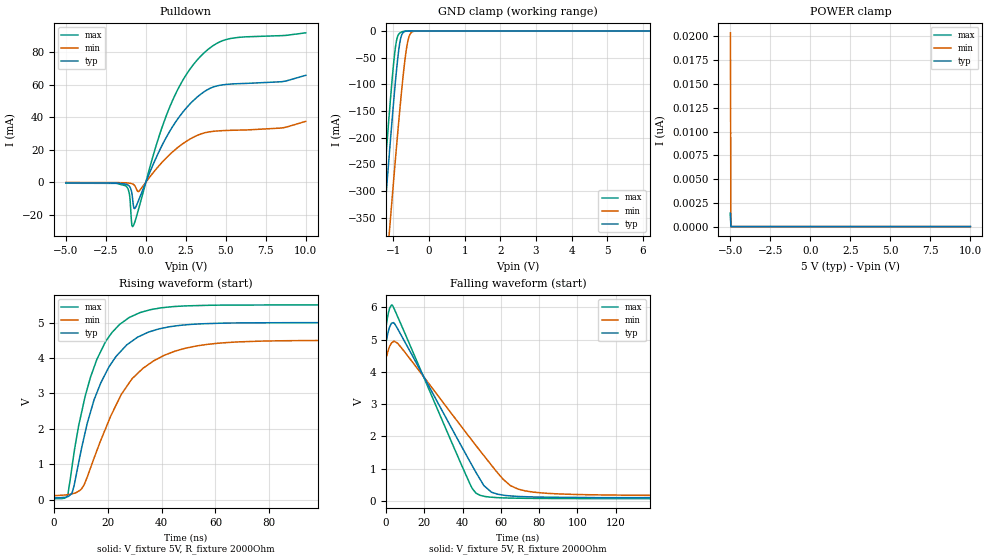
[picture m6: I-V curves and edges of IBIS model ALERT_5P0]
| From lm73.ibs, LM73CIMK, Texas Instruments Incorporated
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|   Model ALERT_5P0
[Model]   ALERT_5P0
Model_type   Open_drain
Polarity   Non-Inverting
Vmeas = 2.5
Vref = 5
Cref = 1pF
Rref = 2000
|   typ   min   max
|   (nom PVT)   (fast PVT)   (slow PVT)
C_comp   0.602p   0.543p   0.661p
|C_comp (ON state)   0.733p   0.730p   0.750p
|C_comp (OFF state)   0.602p   0.543p   0.661p
[Voltage Range]   5   4.5   5.5
[Temperature Range]   27   150   -40
[Pullup Reference]   5   4.5   5.5
[Pulldown Reference]   0   0   0
[Power Clamp Reference]   5   4.5   5.5
[GND Clamp Reference]   0   0   0
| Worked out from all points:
|   slope of the pulldown table from 0 to 0.75 V, typ, clamps not added: 43.3 ohm
|   GND clamp passes 1 mA (typ) near -0.68 V on its own axis
|   falling waveform, V_fixture 5V, R_fixture 2000Ohm: 20-80 % time 27ns typ, 33.7ns min, 23.6ns max; typ from 5 V to 0.097 V
|   rising waveform, V_fixture 5V, R_fixture 2000Ohm: 20-80 % time 13.6ns typ, 17.8ns min, 11.7ns max; typ from 0.097 V to 5 V
[Pulldown]
|   Voltage   I(typ)   I(min)   I(max)
-5V       -394uA     -141.8uA   -589.2uA
-1.25V    -1.146mA   -337.7uA   -2.189mA
-1.025V   -2.466mA   -540.2uA   -7.273mA
-890mV    -5.802mA   -809.4uA   -24.79mA
-815mV    -11.12mA   -1.087mA   -27.23mA
-665mV    -15.89mA   -2.513mA   -23.81mA
-425mV    -10.48mA   -5.487mA   -15.58mA
1.315V    28.32mA    15.36mA    41.94mA
2.32V     43.27mA    23.8mA     62.97mA
3.25V     52.8mA     29.03mA    75.76mA
5.05V     60.29mA    31.92mA    88mA
10V       65.91mA    37.54mA    92.06mA
[GND Clamp]
|   Voltage   I(typ)   I(min)   I(max)
-5V       -3.718A    -3.697A    -3.742A
-1.355V   -440.9mA   -580.8mA   -368mA
-1.25V    -349.5mA   -492.9mA   -274.4mA
-1.13V    -247.1mA   -393.7mA   -170.6mA
-1.07V    -197.3mA   -344.8mA   -121.2mA
-920mV    -81.51mA   -225.7mA   -22.09mA
-830mV    -27.93mA   -157.8mA   -4.69mA
-755mV    -6.077mA   -104.9mA   -1.502mA
-665mV    -667.7uA   -50.27mA   -221.1uA
-590mV    -95.28uA   -18.6mA    -27.79uA
-410mV    -439.3nA   -358.3uA   -36.45nA
10V       0A         0A         0A
[POWER Clamp]
|   Voltage   I(typ)   I(min)   I(max)
-5V       1.395nA    20.39nA    1.449nA
-4.97V    0A         0A         0A
-4.955V   0A         0A         0A
10V       0A         0A         0A
[Ramp]
R_load = 2000
|   typ   min   max
dV/dt_r   2.94209/1.35708e-08   2.60241/1.77746e-08   3.25792/1.17012e-08
dV/dt_f   2.94171/2.70212e-08   2.60108/3.36912e-08   3.2578/2.36341e-08
[Falling Waveform]
V_fixture = 5V
V_fixture_min = 4.5V
V_fixture_max = 5.5V
R_fixture = 2000Ohm
C_fixture = 0F
|   Time   V(typ)   V(min)   V(max)
0s        5V         4.5V       5.5V
1.801ns   5.386V     4.786V     5.966V
3.497ns   5.52V      4.927V     6.044V
8.162ns   5.106V     4.732V     5.423V
43.97ns   1.205V     1.949V     511.1mV
49.07ns   678.6mV    1.559V     176.5mV
55.11ns   269.9mV    1.105V     115.6mV
65ns      156.5mV    474.8mV    89.61mV
73ns      131.8mV    309.7mV    82.22mV
199.9ns   97.15mV    164.9mV    70.34mV
[Rising Waveform]
V_fixture = 5V
V_fixture_min = 4.5V
V_fixture_max = 5.5V
R_fixture = 2000Ohm
C_fixture = 0F
|   Time   V(typ)   V(min)   V(max)
0s        96.53mV    162.6mV    70.16mV
5.233ns   91.24mV    145mV      155.5mV
6.823ns   209.3mV    169.3mV    973.6mV
9.216ns   1.05V      244.2mV    2.089V
16ns      3.024V     1.392V     3.966V
25.07ns   4.208V     2.977V     4.985V
31.97ns   4.621V     3.629V     5.283V
45ns      4.905V     4.196V     5.456V
65ns      4.988V     4.442V     5.495V
199.9ns   5V         4.5V       5.5V
